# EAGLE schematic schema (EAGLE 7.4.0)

## Sheet 1 of 2: SHEEY FSDFSF
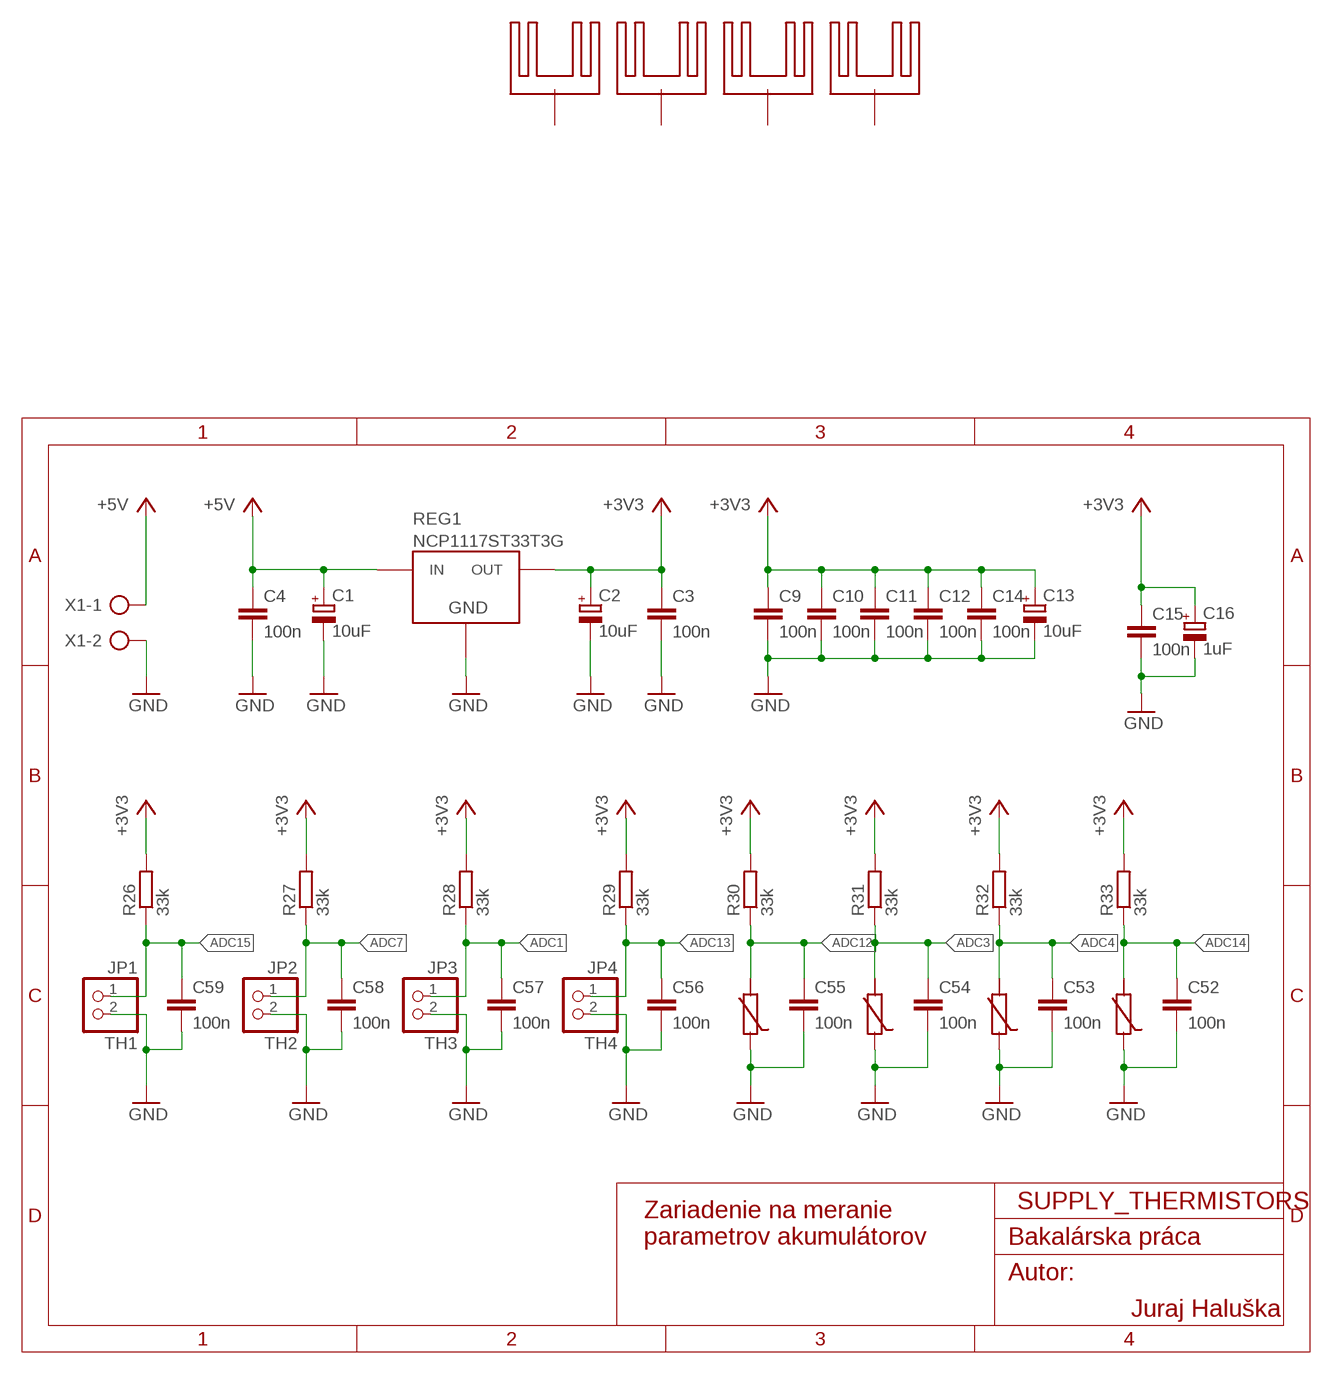
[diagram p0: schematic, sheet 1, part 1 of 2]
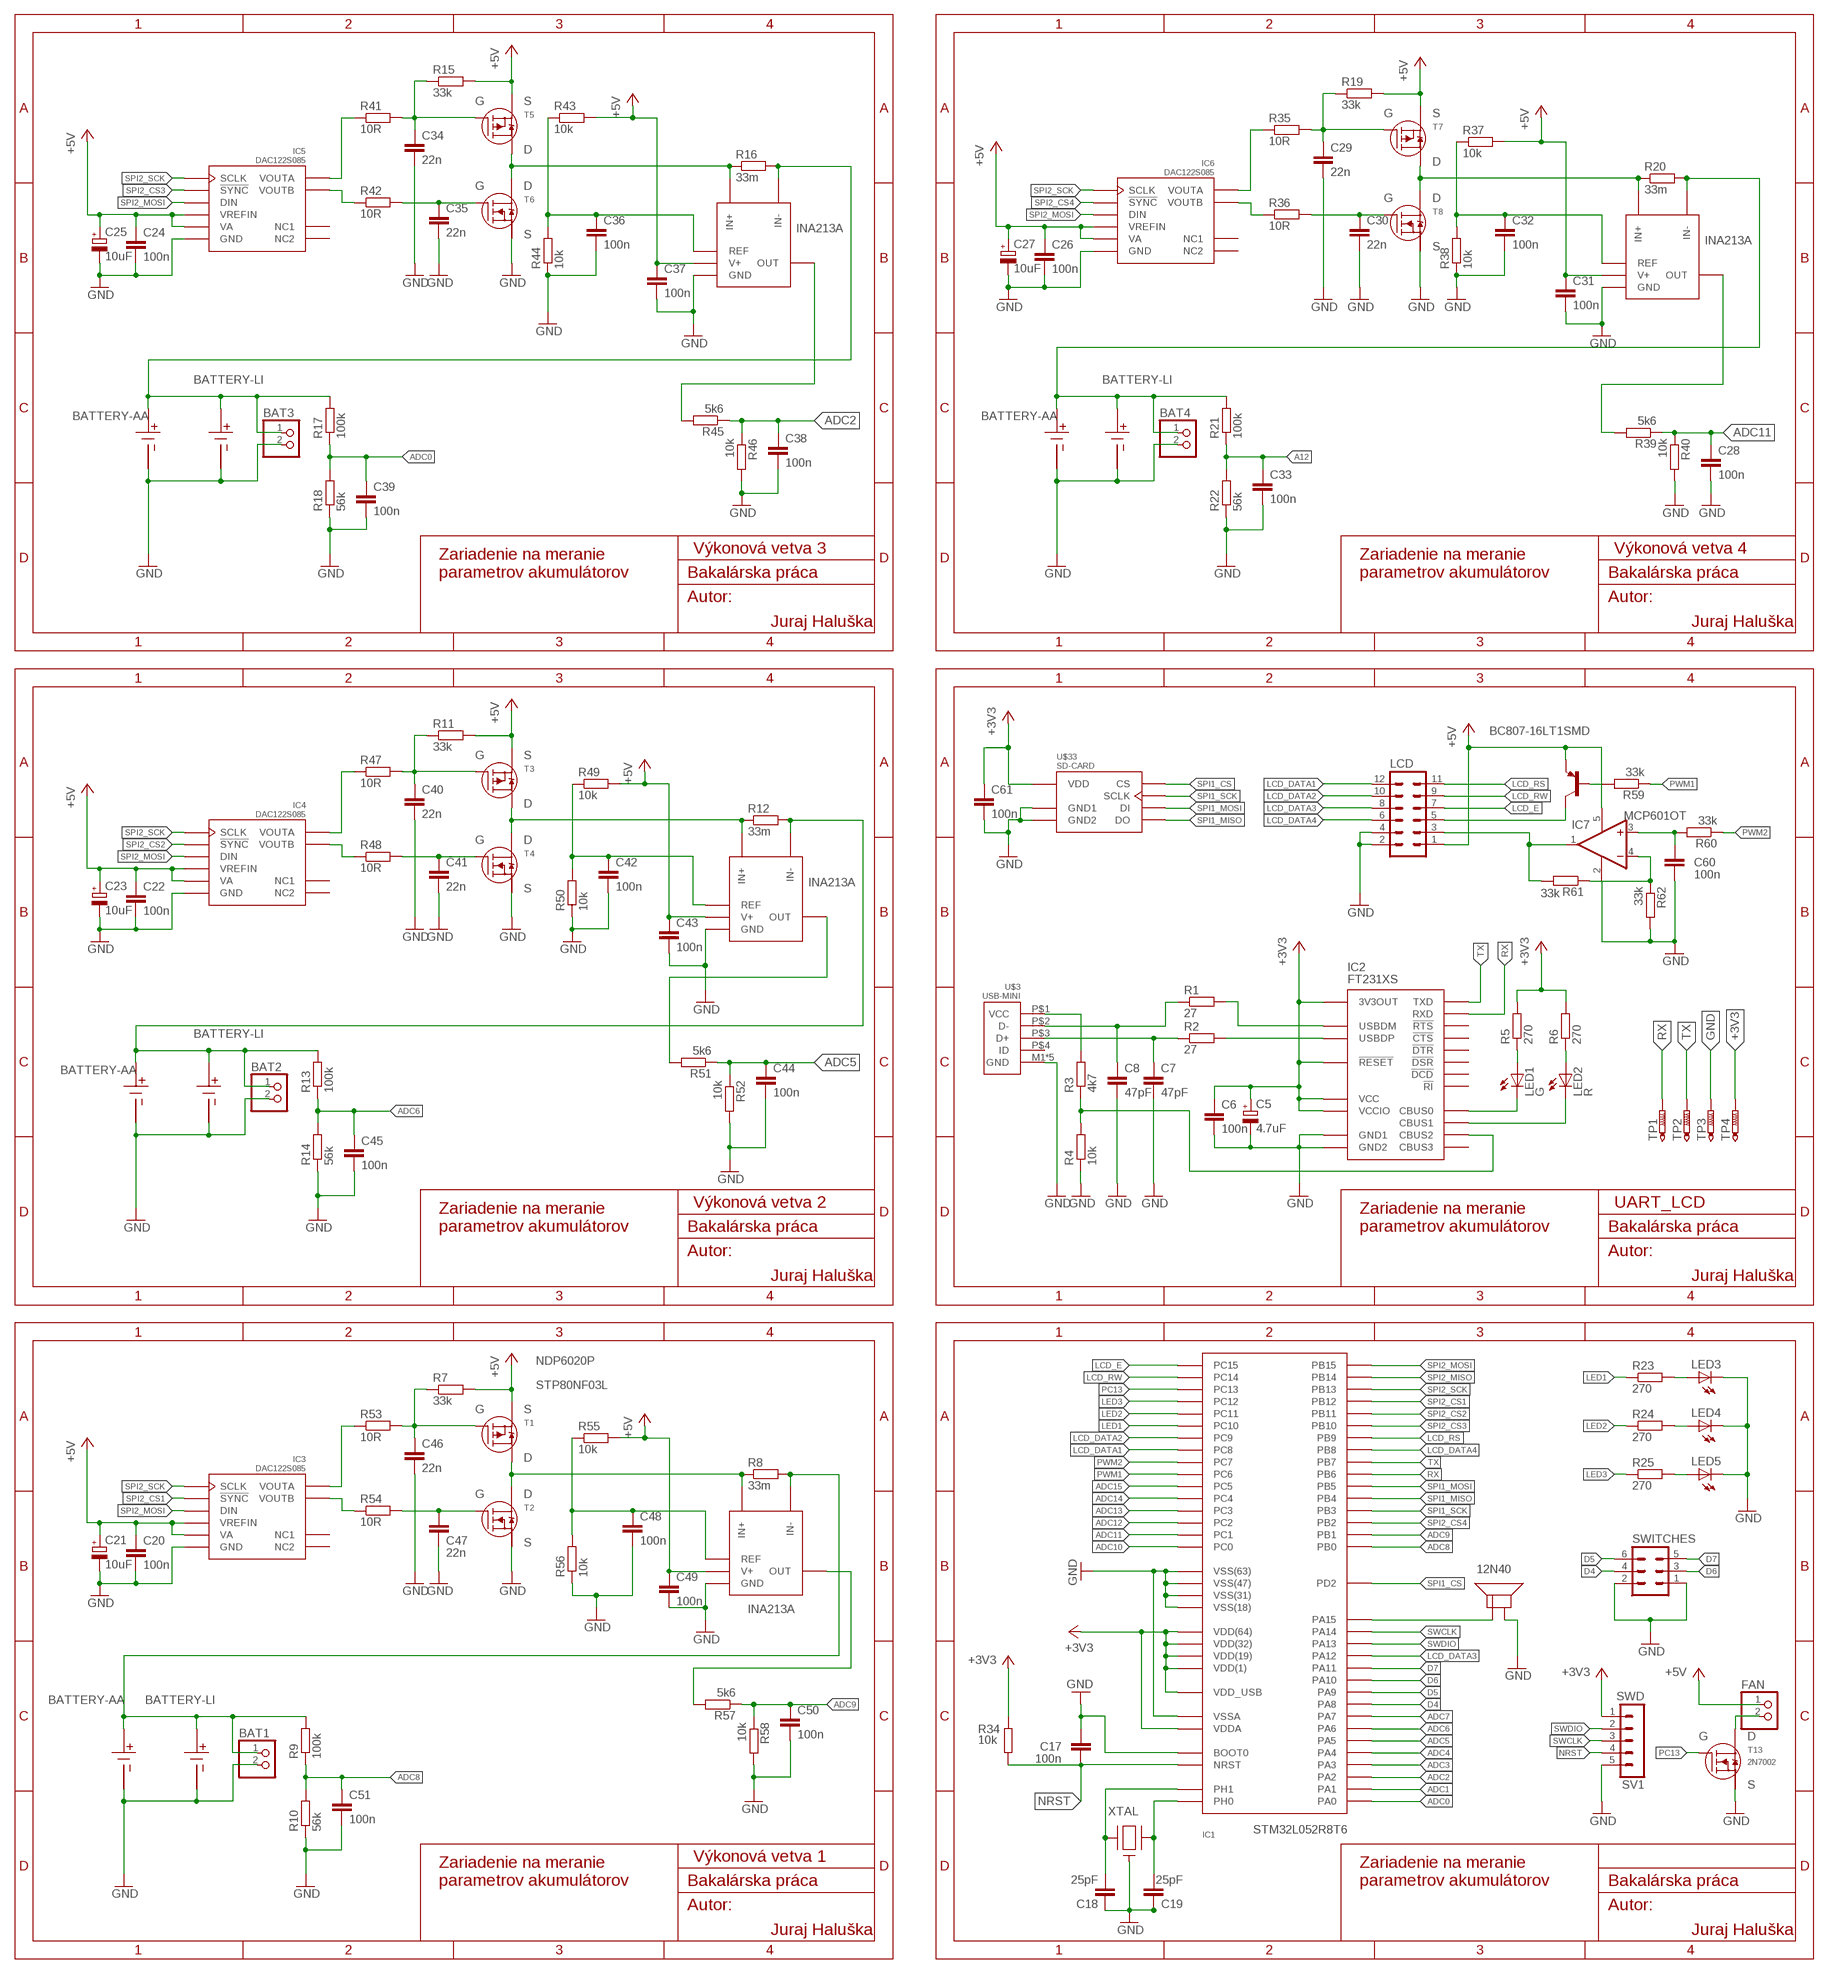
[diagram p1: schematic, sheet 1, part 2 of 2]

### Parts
B1  BATTERY-LI  [KEYSTONE1042]
B2  BATTERY-LI  [KEYSTONE1042]
B3  BATTERY-LI  [KEYSTONE1042]
B4  BATTERY-LI  [KEYSTONE1042]
BAT1  PINHD-1X2  [1X02]
BAT2  PINHD-1X2  [1X02]
BAT3  PINHD-1X2  [1X02]
BAT4  PINHD-1X2  [1X02]
C1  10uF  C-B  [SMDB]
C2  10uF  C-B  [SMDB]
C3  100n  C-0805  [SMD0805C]
C4  100n  C-0805  [SMD0805C]
C5  4.7uF  C-B  [SMDB]
C6  100n  C-0805  [SMD0805C]
C7  47pF  C-0805  [SMD0805C]
C8  47pF  C-0805  [SMD0805C]
C9  100n  C-0805  [SMD0805C]
C10  100n  C-0805  [SMD0805C]
C11  100n  C-0805  [SMD0805C]
C12  100n  C-0805  [SMD0805C]
C13  10uF  C-B  [SMDB]
C14  100n  C-0805  [SMD0805C]
C15  100n  C-0805  [SMD0805C]
C16  1uF  C-B  [SMDB]
C17  100n  C-0805  [SMD0805C]
C18  25pF  C-0805  [SMD0805C]
C19  25pF  C-0805  [SMD0805C]
C20  100n  C-0805  [SMD0805C]
C21  10uF  C-B  [SMDB]
C22  100n  C-0805  [SMD0805C]
C23  10uF  C-B  [SMDB]
C24  100n  C-0805  [SMD0805C]
C25  10uF  C-B  [SMDB]
C26  100n  C-0805  [SMD0805C]
C27  10uF  C-B  [SMDB]
C28  100n  C-0805  [SMD0805C]
C29  22n  C-0805  [SMD0805C]
C30  22n  C-0805  [SMD0805C]
C31  100n  C-0805  [SMD0805C]
C32  100n  C-0805  [SMD0805C]
C33  100n  C-0805  [SMD0805C]
C34  22n  C-0805  [SMD0805C]
C35  22n  C-0805  [SMD0805C]
C36  100n  C-0805  [SMD0805C]
C37  100n  C-0805  [SMD0805C]
C38  100n  C-0805  [SMD0805C]
C39  100n  C-0805  [SMD0805C]
C40  22n  C-0805  [SMD0805C]
C41  22n  C-0805  [SMD0805C]
C42  100n  C-0805  [SMD0805C]
C43  100n  C-0805  [SMD0805C]
C44  100n  C-0805  [SMD0805C]
C45  100n  C-0805  [SMD0805C]
C46  22n  C-0805  [SMD0805C]
C47  22n  C-0805  [SMD0805C]
C48  100n  C-0805  [SMD0805C]
C49  100n  C-0805  [SMD0805C]
C50  100n  C-0805  [SMD0805C]
C51  100n  C-0805  [SMD0805C]
C52  100n  C-0805  [SMD0805C]
C53  100n  C-0805  [SMD0805C]
C54  100n  C-0805  [SMD0805C]
C55  100n  C-0805  [SMD0805C]
C56  100n  C-0805  [SMD0805C]
C57  100n  C-0805  [SMD0805C]
C58  100n  C-0805  [SMD0805C]
C59  100n  C-0805  [SMD0805C]
C60  100n  C-0805  [SMD0805C]
C61  100n  C-0805  [SMD0805C]
FAN  PINHD-1X2  [1X02]
IC1  STM32L052X6/8  [LQFP64]
IC2  FT231XS  [SSOP20]
IC3  DAC122S085  [VSSOP]
IC4  DAC122S085  [VSSOP]
IC5  DAC122S085  [VSSOP]
IC6  DAC122S085  [VSSOP]
IC7  MCP601OT  [SOT23-5]
JP1  TH1  PINHD-1X2  [1X02]
JP2  TH2  PINHD-1X2  [1X02]
JP3  TH3  PINHD-1X2  [1X02]
JP4  TH4  PINHD-1X2  [1X02]
LCD  MA06-2  [MA06-2]
LED1  G  LEDSML0805  [SML0805]
LED2  R  LEDSML0805  [SML0805]
LED3  LEDSML0805  [SML0805]
LED4  LEDSML0805  [SML0805]
LED5  LEDSML0805  [SML0805]
Q1  BC807-16LT1SMD  [SOT23-BEC]
R1  27  R-0805  [SMD0805R]
R2  27  R-0805  [SMD0805R]
R3  4k7  R-0805  [SMD0805R]
R4  10k  R-0805  [SMD0805R]
R5  270  R-0805  [SMD0805R]
R6  270  R-0805  [SMD0805R]
R7  33k  R-0805  [SMD0805R]
R8  33m  RSENSE  [CURRENT_SENSE]
R9  100k  R-0805  [SMD0805R]
R10  56k  R-0805  [SMD0805R]
R11  33k  R-0805  [SMD0805R]
R12  33m  RSENSE  [CURRENT_SENSE]
R13  100k  R-0805  [SMD0805R]
R14  56k  R-0805  [SMD0805R]
R15  33k  R-0805  [SMD0805R]
R16  33m  RSENSE  [CURRENT_SENSE]
R17  100k  R-0805  [SMD0805R]
R18  56k  R-0805  [SMD0805R]
R19  33k  R-0805  [SMD0805R]
R20  33m  RSENSE  [CURRENT_SENSE]
R21  100k  R-0805  [SMD0805R]
R22  56k  R-0805  [SMD0805R]
R23  270  R-0805  [SMD0805R]
R24  270  R-0805  [SMD0805R]
R25  270  R-0805  [SMD0805R]
R26  33k  R-0805  [SMD0805R]
R27  33k  R-0805  [SMD0805R]
R28  33k  R-0805  [SMD0805R]
R29  33k  R-0805  [SMD0805R]
R30  33k  R-0805  [SMD0805R]
R31  33k  R-0805  [SMD0805R]
R32  33k  R-0805  [SMD0805R]
R33  33k  R-0805  [SMD0805R]
R34  10k  R-0805  [SMD0805R]
R35  10R  R-0805  [SMD0805R]
R36  10R  R-0805  [SMD0805R]
R37  10k  R-0805  [SMD0805R]
R38  10k  R-0805  [SMD0805R]
R39  5k6  R-0805  [SMD0805R]
R40  10k  R-0805  [SMD0805R]
R41  10R  R-0805  [SMD0805R]
R42  10R  R-0805  [SMD0805R]
R43  10k  R-0805  [SMD0805R]
R44  10k  R-0805  [SMD0805R]
R45  5k6  R-0805  [SMD0805R]
R46  10k  R-0805  [SMD0805R]
R47  10R  R-0805  [SMD0805R]
R48  10R  R-0805  [SMD0805R]
R49  10k  R-0805  [SMD0805R]
R50  10k  R-0805  [SMD0805R]
R51  5k6  R-0805  [SMD0805R]
R52  10k  R-0805  [SMD0805R]
R53  10R  R-0805  [SMD0805R]
R54  10R  R-0805  [SMD0805R]
R55  10k  R-0805  [SMD0805R]
R56  10k  R-0805  [SMD0805R]
R57  5k6  R-0805  [SMD0805R]
R58  10k  R-0805  [SMD0805R]
R59  33k  R-0805  [SMD0805R]
R60  33k  R-0805  [SMD0805R]
R61  33k  R-0805  [SMD0805R]
R62  33k  R-0805  [SMD0805R]
REG1  NCP1117ST33T3G  [SOT223]
SV1  SWD  MA05-1  [MA05-1]
SWITCHES  MA03-2  [MA03-2]
T1  NDP6020P  [TO220]
T2  STP80NF03L-04  [TO220]
T3  NDP6020P  [TO220]
T4  STP80NF03L-04  [TO220]
T5  NDP6020P  [TO220]
T6  STP80NF03L-04  [TO220]
T7  NDP6020P  [TO220]
T8  STP80NF03L-04  [TO220]
T13  2N7002  [SOT23]
TP1  PTR1B1,27  [B1,27]
TP2  PTR1B1,27  [B1,27]
TP3  PTR1B1,27  [B1,27]
TP4  PTR1B1,27  [B1,27]
U$1  XTAL  [XTAL-TSX-3225]
U$2  INA213A  [DCK(INA213)]
U$3  USB-MINI  [USB-MINI]
U$4  INA213A  [DCK(INA213)]
U$5  INA213A  [DCK(INA213)]
U$6  INA213A  [DCK(INA213)]
U$9  THERMISTOR  [THERMISTOR]
U$10  THERMISTOR  [THERMISTOR]
U$11  BATTERY-AA  [KEYSTONE1015]
U$12  THERMISTOR  [THERMISTOR]
U$15  THERMISTOR  [THERMISTOR]
U$16  CHLADIC  [CHLADIC]
U$17  CHLADIC  [CHLADIC]
U$18  BATTERY-AA  [KEYSTONE1015]
U$19  CHLADIC  [CHLADIC]
U$22  CHLADIC  [CHLADIC]
U$25  BATTERY-AA  [KEYSTONE1015]
U$32  BATTERY-AA  [KEYSTONE1015]
U$33  SD-CARD  [SD-SOCKET]
U$34  12N40  [12N40]
X1  AK500/2-H  [AK500/2-H]

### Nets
+3V3: C2.P$1(+) C3.P$1 C5.P$1(+) C6.P$1 C9.P$1 C10.P$1 C11.P$1 C12.P$1 C13.P$1(+) C14.P$1 C15.P$1 C16.P$1(+) C61.P$1 IC1.P$1(VDD(1)) IC1.P$13(VDDA) IC1.P$19(VDD(19)) IC1.P$32(VDD(32)) IC1.P$48(VDD_USB) IC1.P$64(VDD(64)) IC2.P$3(VCCIO) IC2.P$13(3V3OUT) IC2.P$14(!RESET) IC2.P$15(VCC) R5.P$2 R6.P$2 R26.P$2 R27.P$2 R28.P$2 R29.P$2 R30.P$2 R31.P$2 R32.P$2 R33.P$2 R34.P$2 REG1.P$2(OUT) REG1.P$4(OUT) SV1.1 TP4.TP U$33.P$4(VDD)
+5V: C1.P$1(+) C4.P$1 C20.P$1 C21.P$1(+) C22.P$1 C23.P$1(+) C24.P$1 C25.P$1(+) C26.P$1 C27.P$1(+) C31.P$1 C37.P$1 C43.P$1 C49.P$1 FAN.1 IC3.P$1(VA) IC3.P$7(VREFIN) IC4.P$1(VA) IC4.P$7(VREFIN) IC5.P$1(VA) IC5.P$7(VREFIN) IC6.P$1(VA) IC6.P$7(VREFIN) IC7.5(V+) LCD.1 Q1.E R7.P$2 R11.P$2 R15.P$2 R19.P$2 R37.P$2 R43.P$2 R49.P$2 R55.P$2 REG1.P$3(IN) T1.P$3 T3.P$3 T5.P$3 T7.P$3 U$2.P$3(V+) U$4.P$3(V+) U$5.P$3(V+) U$6.P$3(V+) X1.1
A12: C33.P$1 R21.P$1 R22.P$2
ADC0: C39.P$1 IC1.P$14(PA0) R17.P$1 R18.P$2
ADC1: C57.P$1 IC1.P$15(PA1) JP3.1 R28.P$1
ADC2: C38.P$1 IC1.P$16(PA2) R45.P$1 R46.P$1
ADC3: C54.P$1 IC1.P$17(PA3) R31.P$1 U$10.2
ADC4: C53.P$1 IC1.P$20(PA4) R32.P$1 U$12.2
ADC5: C44.P$1 IC1.P$21(PA5) R51.P$1 R52.P$1
ADC6: C45.P$1 IC1.P$22(PA6) R13.P$1 R14.P$2
ADC7: C58.P$1 IC1.P$23(PA7) JP2.1 R27.P$1
ADC8: C51.P$1 IC1.P$26(PB0) R9.P$1 R10.P$2
ADC9: C50.P$1 IC1.P$27(PB1) R57.P$1 R58.P$1
ADC10: IC1.P$8(PC0)
ADC11: C28.P$1 IC1.P$9(PC1) R39.P$1 R40.P$1
ADC12: C55.P$1 IC1.P$10(PC2) R30.P$1 U$9.2
ADC13: C56.P$1 IC1.P$11(PC3) JP4.1 R29.P$1
ADC14: C52.P$1 IC1.P$24(PC4) R33.P$1 U$15.2
ADC15: C59.P$1 IC1.P$25(PC5) JP1.1 R26.P$1
D4: IC1.P$41(PA8) SWITCHES.4
D5: IC1.P$42(PA9) SWITCHES.6
D6: IC1.P$43(PA10) SWITCHES.3
D7: IC1.P$44(PA11) SWITCHES.5
GND: B1.P$1(MINUS) B2.P$1(MINUS) B3.P$1(MINUS) B4.P$1(MINUS) BAT1.2 BAT2.2 BAT3.2 BAT4.2 C1.P$2(-) C2.P$2(-) C3.P$2 C4.P$2 C5.P$2(-) C6.P$2 C7.P$2 C8.P$2 C9.P$2 C10.P$2 C11.P$2 C12.P$2 C13.P$2(-) C14.P$2 C15.P$2 C16.P$2(-) C17.P$2 C18.P$1 C19.P$1 C20.P$2 C21.P$2(-) C22.P$2 C23.P$2(-) C24.P$2 C25.P$2(-) C26.P$2 C27.P$2(-) C28.P$2 C29.P$2 C30.P$2 C31.P$2 C32.P$2 C33.P$2 C34.P$2 C35.P$2 C36.P$2 C37.P$2 C38.P$2 C39.P$2 C40.P$2 C41.P$2 C42.P$2 C43.P$2 C44.P$2 C45.P$2 C46.P$2 C47.P$2 C48.P$2 C49.P$2 C50.P$2 C51.P$2 C52.P$2 C53.P$2 C54.P$2 C55.P$2 C56.P$2 C57.P$2 C58.P$2 C59.P$2 C60.P$2 C61.P$2 IC1.P$12(VSSA) IC1.P$18(VSS(18)) IC1.P$31(VSS(31)) IC1.P$47(VSS(47)) IC1.P$60(BOOT0) IC1.P$63(VSS(63)) IC2.P$6(GND1) IC2.P$16(GND2) IC3.P$6(GND) IC4.P$6(GND) IC5.P$6(GND) IC6.P$6(GND) IC7.2(V-) JP1.2 JP2.2 JP3.2 JP4.2 LCD.2 LCD.4 LED3.C LED4.C LED5.C R4.P$1 R10.P$1 R14.P$1 R18.P$1 R22.P$1 R38.P$1 R40.P$2 R44.P$1 R46.P$2 R50.P$1 R52.P$2 R56.P$1 R58.P$2 R62.P$2 REG1.P$1(GND) SV1.5 SWITCHES.1 SWITCHES.2 T2.P$3(SOURCE) T4.P$3(SOURCE) T6.P$3(SOURCE) T8.P$3(SOURCE) T13.2(SOURCE) TP3.TP U$1.GND1(GND) U$1.GND2(GND) U$2.P$2(GND) U$3.M1(GND) U$3.M2(GND) U$3.M3(GND) U$3.M4(GND) U$3.P$5(GND) U$4.P$2(GND) U$5.P$2(GND) U$6.P$2(GND) U$9.1 U$10.1 U$11.P$1(MINUS) U$12.1 U$15.1 U$18.P$1(MINUS) U$25.P$1(MINUS) U$32.P$1(MINUS) U$33.DC(GND1) U$33.GND(GND1) U$33.M1(GND1) U$33.M2(GND1) U$33.OPT(GND1) U$33.P$3(GND1) U$33.P$6(GND2) U$33.WP(GND1) U$34.P$2(MINUS) X1.2
LCD_DATA1: IC1.P$39(PC8) LCD.12
LCD_DATA2: IC1.P$40(PC9) LCD.10
LCD_DATA3: IC1.P$45(PA12) LCD.8
LCD_DATA4: IC1.P$61(PB8) LCD.6
LCD_E: IC1.P$4(PC15) LCD.7
LCD_RS: IC1.P$62(PB9) LCD.11
LCD_RW: IC1.P$3(PC14) LCD.9
LED1: IC1.P$51(PC10) R23.P$1
LED2: IC1.P$52(PC11) R24.P$1
LED3: IC1.P$53(PC12) R25.P$1
N$1: IC2.P$12(USBDM) R1.P$2
N$2: C19.P$2 IC1.P$5(PH0) U$1.P$2
N$3: C8.P$1 R1.P$1 U$3.P$2(D-)
N$4: C7.P$1 R2.P$1 U$3.P$3(D+)
N$5: IC2.P$11(USBDP) R2.P$2
N$6: C18.P$2 IC1.P$6(PH1) U$1.P$4
N$7: IC2.P$10(CBUS2) R3.P$1 R4.P$2
N$8: R3.P$2 U$3.P$1(VCC)
N$9: IC6.P$2(VOUTA) R35.P$1
N$10: IC2.P$18(CBUS0) LED1.C
N$11: IC2.P$17(CBUS1) LED2.C
N$12: LED1.A R5.P$1
N$13: LED2.A R6.P$1
N$14: C29.P$1 R19.P$1 R35.P$2 T7.P$1
N$15: C46.P$1 R7.P$1 R53.P$2 T1.P$1
N$16: IC6.P$3(VOUTB) R36.P$1
N$17: IC3.P$3(VOUTB) R54.P$1
N$18: R8.P$1 T1.P$2 T2.P$2(DRAIN) U$6.P$4(IN+)
N$19: B4.P$2(PLUS) BAT1.1 R8.P$2 R9.P$2 U$6.P$5(IN-) U$11.P$2(PLUS)
N$20: C30.P$1 R36.P$2 T8.P$1(GATE)
N$21: C32.P$1 R37.P$1 R38.P$2 U$2.P$1(REF)
N$22: C40.P$1 R11.P$1 R47.P$2 T3.P$1
N$23: R39.P$2 U$2.P$6(OUT)
N$24: IC4.P$3(VOUTB) R48.P$1
N$25: R12.P$1 T3.P$2 T4.P$2(DRAIN) U$5.P$4(IN+)
N$26: B3.P$2(PLUS) BAT2.1 R12.P$2 R13.P$2 U$5.P$5(IN-) U$18.P$2(PLUS)
N$27: IC1.P$50(PA15) U$34.P$1(PLUS)
N$28: IC5.P$2(VOUTA) R41.P$1
N$29: C34.P$1 R15.P$1 R41.P$2 T5.P$1
N$30: C35.P$1 R42.P$2 T6.P$1(GATE)
N$31: IC5.P$3(VOUTB) R42.P$1
N$32: R16.P$1 T5.P$2 T6.P$2(DRAIN) U$4.P$4(IN+)
N$33: B1.P$2(PLUS) BAT3.1 R16.P$2 R17.P$2 U$4.P$5(IN-) U$25.P$2(PLUS)
N$34: C36.P$1 R43.P$1 R44.P$2 U$4.P$1(REF)
N$35: IC4.P$2(VOUTA) R47.P$1
N$36: C41.P$1 R48.P$2 T4.P$1(GATE)
N$37: R45.P$2 U$4.P$6(OUT)
N$38: C42.P$1 R49.P$1 R50.P$2 U$5.P$1(REF)
N$41: LED3.A R23.P$2
N$42: LED4.A R24.P$2
N$43: LED5.A R25.P$2
N$44: Q1.B R59.P$2
N$45: FAN.2 T13.3(DRAIN)
N$46: R51.P$2 U$5.P$6(OUT)
N$47: C47.P$1 R54.P$2 T2.P$1(GATE)
N$48: IC3.P$2(VOUTA) R53.P$1
N$49: C48.P$1 R55.P$1 R56.P$2 U$6.P$1(REF)
N$50: R57.P$2 U$6.P$6(OUT)
N$51: LCD.5 Q1.C
N$52: C60.P$1 IC7.3(+IN) R60.P$2
N$53: IC7.1(OUT) LCD.3 R61.P$2
N$56: IC7.4(-IN) R61.P$1 R62.P$1
N$99: B2.P$2(PLUS) BAT4.1 R20.P$2 R21.P$2 U$2.P$5(IN-) U$32.P$2(PLUS)
NRST: C17.P$1 IC1.P$7(NRST) R34.P$1 SV1.4
PC13: IC1.P$2(PC13) T13.1(GATE)
PWM1: IC1.P$37(PC6) R59.P$1
PWM2: IC1.P$38(PC7) R60.P$1
RX: IC1.P$58(PB6) IC2.P$4(RXD) TP1.TP
SPI1_CS: IC1.P$54(PD2) U$33.P$1(CS)
SPI1_MISO: IC1.P$56(PB4) U$33.P$7(DO)
SPI1_MOSI: IC1.P$57(PB5) U$33.P$2(DI)
SPI1_SCK: IC1.P$55(PB3) U$33.P$5(SCLK)
SPI2_CS1: IC1.P$33(PB12) IC3.P$9(!SYNC)
SPI2_CS2: IC1.P$30(PB11) IC4.P$9(!SYNC)
SPI2_CS3: IC1.P$29(PB10) IC5.P$9(!SYNC)
SPI2_CS4: IC1.P$28(PB2) IC6.P$9(!SYNC)
SPI2_MISO: IC1.P$35(PB14)
SPI2_MOSI: IC1.P$36(PB15) IC3.P$8(DIN) IC4.P$8(DIN) IC5.P$8(DIN) IC6.P$8(DIN)
SPI2_SCK: IC1.P$34(PB13) IC3.P$10(SCLK) IC4.P$10(SCLK) IC5.P$10(SCLK) IC6.P$10(SCLK)
SWCLK: IC1.P$49(PA14) SV1.3
SWDIO: IC1.P$46(PA13) SV1.2
T: R20.P$1 T7.P$2 T8.P$2(DRAIN) U$2.P$4(IN+)
TX: IC1.P$59(PB7) IC2.P$20(TXD) TP2.TP
Unconnected: IC2.P$1(!DTR) IC2.P$2(!RTS) IC2.P$5(!RI) IC2.P$7(!DSR) IC2.P$8(!DCD) IC2.P$9(!CTS) IC2.P$19(CBUS3) IC3.P$4(NC1) IC3.P$5(NC2) IC4.P$4(NC1) IC4.P$5(NC2) IC5.P$4(NC1) IC5.P$5(NC2) IC6.P$4(NC1) IC6.P$5(NC2) U$3.P$4(ID) U$16.P$1 U$16.P$2 U$16.P$4 U$17.P$1 U$17.P$2 U$17.P$4 U$19.P$1 U$19.P$2 U$19.P$4 U$22.P$1 U$22.P$2 U$22.P$4

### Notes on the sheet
- Výkonová vetva 3 | Výkonová vetva 4
- SUPPLY_THERMISTORS
- Výkonová vetva 2 | UART_LCD
- NDP6020P
- STP80NF03L
- STM32L052R8T6
- Výkonová vetva 1

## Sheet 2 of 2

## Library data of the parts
B1-B4 = suciastky:BATTERY-LI
BAT1-BAT4 FAN JP1-JP4 = pinhead:PINHD-1X2: PIN HEADER
C1 C2 C5 C13 C16 C21 C23 C25 C27 = suciastky:C-B
C3 C4 C6-C12 C14 C15 C17-C20 C22 C24 C26 C28-C61 = suciastky:C-0805
IC1 = suciastky:STM32L052X6/8
IC2 = suciastky:FT231XS
IC3-IC6 = suciastky:DAC122S085
IC7 = linear:MCP601: Single Op Amp 2.7V to 6.0V Single Supply CMOS Source: http://ww1.microchip.com/downloads/en/DeviceDoc/21314g.pdf
LCD = con-lstb:MA06-2: PIN HEADER; OC_FARNELL: unknown; OC_NEWARK: unknown
LED1-LED5 = led:LED: LED
Q1 = transistor-pnp:BC807*: PNP Transistror
R1-R7 R9-R11 R13-R15 R17-R19 R21-R62 = suciastky:R-0805
R8 R12 R16 R20 = suciastky:RSENSE
REG1 = suciastky:NCP1117ST33T3G
SV1 = con-lstb:MA05-1: PIN HEADER; OC_FARNELL: unknown; OC_NEWARK: unknown
SWITCHES = con-lstb:MA03-2: PIN HEADER; OC_FARNELL: unknown; OC_NEWARK: unknown
T1 T3 T5 T7 = suciastky:NDP6020P
T2 T4 T6 T8 = suciastky:STP80NF03L-04
T13 = suciastky:2N7002
TP1-TP4 = testpad:PTR1: TEST PIN
U$1 = suciastky:XTAL
U$2 U$4-U$6 = suciastky:INA213A
U$3 = suciastky:USB-MINI
U$9 U$10 U$12 U$15 = suciastky:THERMISTOR
U$11 U$18 U$25 U$32 = suciastky:BATTERY-AA
U$16 U$17 U$19 U$22 = suciastky:CHLADIC
U$33 = suciastky:SD-CARD
U$34 = suciastky:12N40
X1 = con-ptr500:AK500/2-H: CONNECTOR; OC_FARNELL: unknown; OC_NEWARK: unknown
